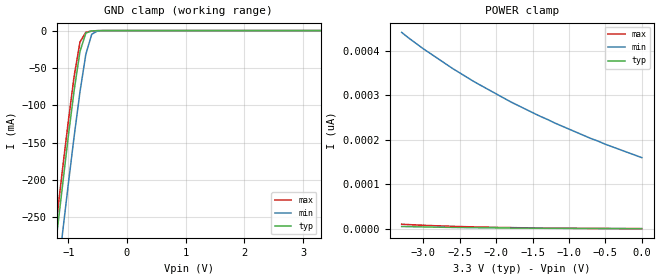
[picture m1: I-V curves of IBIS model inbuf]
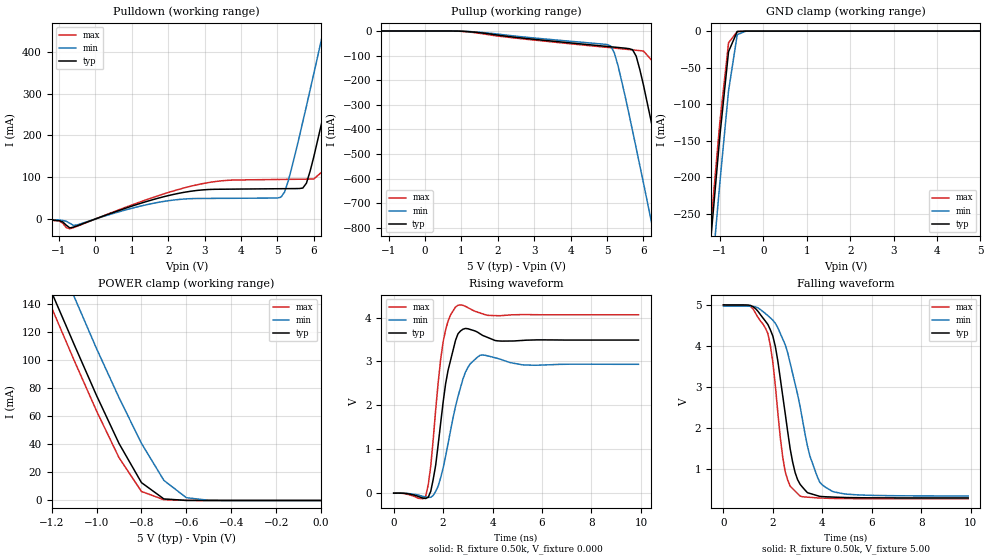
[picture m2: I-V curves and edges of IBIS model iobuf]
| IBIS file 64245l.ibs created by s2ibis2 version 1.0
| North Carolina State University Electronics Research Laboratory  1995
[IBIS ver]   2.1
[File name]   64245l.ibs
[File Rev]   0.1
[Date]   Friday, August 15, 1997
[Source]   IDT
[Notes]   1. Temp typ=25C, min=100C, max=0C 2. Ramp rates based on 500
   ohm load
[Copyright]   Copyright 1997, Integrated Device Technology, Inc.
[Disclaimer] Integrated Device Technology, Inc. ("IDT") hereby grants the
   user of this IBIS model a non-exclusive, nontransferable
   license to use this IBIS model under the following terms.
   The user is granted this license only to use the IBIS model
   and is not granted rights to sell, copy (except as needed to
   run the IBIS model), rent, lease or sub-license the IBIS model
   in whole or in part, or in modified form to anyone.
   The User may modify the IBIS model to suit its specific
   applications, but rights to derivative works and such
   modifications shall belong to IDT.
   This IBIS model is provided on an "AS IS" basis and IDT
   makes absolutely no warranty with respect to the information
   contained herein. IDT DISCLAIMS AND CUSTOMER WAIVES ALL
   WARRANTIES, EXPRESS AND IMPLIED, INCLUDING WARRANTIES OF
   MERCHANTABILITY AND FITNESS FOR A PARTICULAR PURPOSE. THE
   ENTIRE RISK AS TO QUALITY AND PERFORMANCE IS WITH THE
   USER ACCORDINGLY, IN NO EVENT SHALL IDT BE LIABLE
   FOR ANY DIRECT OR INDIRECT DAMAGES, WHETHER IN CONTRACT OR
   TORT, INCLUDING ANY LOST PROFITS OR OTHER INCIDENTAL,
   CONSEQUENTIAL, EXEMPLARY, OR PUNITIVE DAMAGES ARISING OUT OF
   THE USE OR APPLICATION OF THE IBIS model.  Further, IDT
   reserves the right to make changes without notice to any
   product herein to improve reliability, function, or design.
   IDT does not convey any license under patent rights or
   any other intellectual property rights, including those of
   third parties. IDT is not obligated to provide maintenance
   or support for the licensed IBIS model.
|   Component IDT54/74FCT164245/A/C
[Component]   IDT54/74FCT164245/A/C
[Manufacturer]   Integrated Device Technology Inc.
[Package]
| Following package parameters are for SO48-2(TSSOP) package
|[Package]
|| variable   typ   min   max
R_pkg   15.00m   10.00m   20.00m
L_pkg   2.30nh   1.40nh   4.50nH
C_pkg   0.40pF   0.35pF   0.60pF
| Following package parameters are for SO48-1(SSOP), E48-1(CERPAK) packages
|[Package]
|| variable   typ   min   max
|R_pkg   15.00m   10.00m   20.00m
|L_pkg   2.90nH   1.50nH   5.60nH
|C_pkg   0.40pF   0.26pF   0.50pF
[Pin]  signal_name   model_name   R_pin   L_pin   C_pin
1   1DIR   inbuf
2   1B1   iobuf
3   1B2   iobuf
4   GND   GND
5   1B3   iobuf
6   1B4   iobuf
7   VCC   POWER
8   1B5   iobuf
9   1B6   iobuf
10   GND   GND
11   1B7   iobuf
12   1B8   iobuf
13   2B1   iobuf
14   2B2   iobuf
15   GND   GND
16   2B3   iobuf
17   2B4   iobuf
18   VCC   POWER
19   2B5   iobuf
20   2B6   iobuf
21   GND   GND
22   2B7   iobuf
23   2B8   iobuf
24   2DIR   inbuf
25   2OEB   inbuf
26   2A8   iobuf
27   2A7   iobuf
28   GND   GND
29   2A6   iobuf
30   2A5   iobuf
31   VCC   POWER
32   2A4   iobuf
33   2A3   iobuf
34   GND   GND
35   2A2   iobuf
36   2A1   iobuf
37   1A8   iobuf
38   1A7   iobuf
39   GND   GND
40   1A6   iobuf
41   1A5   iobuf
42   VCC   POWER
43   1A4   iobuf
44   1A3   iobuf
45   GND   GND
46   1A2   iobuf
47   1A1   iobuf
48   1OEB   inbuf
| Models and submodels in the file (2): inbuf (Input), iobuf (I/O)
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| in   IN1   dummy_model
| oe   OE1   dummy_model
|   Model inbuf
[Model]   inbuf
Model_type   Input
Vinl =  0.800V
Vinh =  2.000V
C_comp   3.00pF   NA   NA
[Temperature Range]   25.00   100.00   0.000
[Voltage Range]   3.30V   3.00V   3.60V
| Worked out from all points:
|   GND clamp passes 1 mA (typ) near -0.62 V on its own axis
[GND_clamp]
| voltage   I(typ)   I(min)   I(max)
-3.3V     -1.781A    -1.841A    -1.762A
-1.3V     -346mA     -410mA     -324mA
-1.2V     -276mA     -341mA     -255mA
-1.1V     -209mA     -273mA     -187mA
-1V       -142mA     -206mA     -122mA
-900mV    -80.26mA   -142mA     -61.07mA
-800mV    -27.87mA   -81.82mA   -15.26mA
-700mV    -3.289mA   -31.47mA   -2.24mA
-600mV    -480uA     -4.848mA   -551uA
-500mV    -82.77uA   -464uA     -85.69uA
3.3V      588fA      178pA      482fA
[POWER_clamp]
| voltage   I(typ)   I(min)   I(max)
-3.3V     5.432pA    441pA      10.51pA
-3V       4.444pA    404pA      8.155pA
-2.6V     3.398pA    360pA      5.808pA
-2.3V     2.779pA    330pA      4.5pA
-1.8V     1.984pA    285pA      2.938pA
-1.2V     1.325pA    238pA      1.756pA
-700mV    945fA      203pA      1.142pA
0V        588fA      160pA      625fA
|   Model iobuf
[Model]   iobuf
Model_type   I/O
Polarity   Non-Inverting
Enable   Active-High
Vinl =  0.800V
Vinh =  2.000V
C_comp   3.00pF   NA   NA
[Temperature Range]   25.00   100.00   0.000
[Voltage Range]   5.00V   4.50V   5.50V
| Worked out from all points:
|   slope of the pulldown table from 0 to 0.75 V, typ, clamps not added: 32 ohm
|   slope of the pullup table from 0 to 0.75 V, typ, clamps not added: 16.9 kohm
|   GND clamp passes 1 mA (typ) near -0.60 V on its own axis
|   POWER clamp passes 1 mA (typ) near -0.69 V on its own axis
|   rising waveform, R_fixture 0.50k, V_fixture 0.000: 20-80 % time 485ps typ, 669ps min, 420ps max; typ from 0 V to 3.49 V
|   falling waveform, R_fixture 0.50k, V_fixture 5.00: 20-80 % time 708ps typ, 1.04ns min, 535ps max; typ from 5 V to 0.294 V
[Pulldown]
| voltage   I(typ)   I(min)   I(max)
-5V       0A         0A         0A
-1.4V     -1.4mA     -1.2mA     -1.5mA
-700mV    -21.48mA   -10.28mA   -23.37mA
2.4V      63.27mA    47.55mA    73.49mA
5.1V      72.54mA    52.22mA    94.74mA
5.3V      72.68mA    90.95mA    94.95mA
5.8V      85.74mA    270mA      95.45mA
6.4V      298mA      503mA      126mA
6.8V      454mA      660mA      272mA
7.2V      613mA      818mA      428mA
7.6V      772mA      977mA      586mA
10V       1.734A     1.934A     1.549A
[Pullup]
| voltage   I(typ)   I(min)   I(max)
-5V       0A         0A         0A
900mV     -315uA     -296uA     -632uA
5V        -62.63mA   -55.04mA   -66.48mA
5.2V      -65.46mA   -88.64mA   -69.4mA
5.7V      -75.8mA    -405mA     -76.67mA
5.8V      -102mA     -475mA     -78.12mA
6V        -219mA     -617mA     -81.11mA
6.4V      -498mA     -906mA     -148mA
6.8V      -787mA     -1.197A    -417mA
7.2V      -1.079A    -1.49A     -705mA
7.6V      -1.373A    -1.784A    -998mA
10V       -3.151A    -3.558A    -2.774A
[GND_clamp]
| voltage   I(typ)   I(min)   I(max)
-5V       -3.126A    -3.162A    -3.124A
-1.4V     -422mA     -485mA     -404mA
-1.2V     -280mA     -344mA     -261mA
-1V       -144mA     -208mA     -125mA
-800mV    -28.18mA   -82.09mA   -16.01mA
-600mV    -487uA     -4.87mA    -593uA
-400mV    -1.041uA   -20.98uA   -995nA
5V        1.904pA    145uA      2.071pA
[POWER_clamp]
| voltage   I(typ)   I(min)   I(max)
-5V       1.658A     1.682A     1.65A
-1.3V     186mA      220mA      175mA
-1.2V     148mA      182mA      137mA
-1.1V     111mA      145mA      99.7mA
-1V       74.62mA    108mA      63.64mA
-900mV    40.55mA    73.19mA    30.44mA
-800mV    12.71mA    40.62mA    6.427mA
-700mV    1.113mA    14.29mA    552uA
-600mV    55.94uA    1.985mA    66.61uA
-500mV    1.923uA    144uA      3.688uA
0V        1.904pA    260pA      3.223pA
[Ramp]
| variable   typ   min   max
dV/dt_r   2.09/0.49n   1.76/0.67n   2.44/0.42n
dV/dt_f   2.82/0.71n   2.52/1.02n   3.12/0.54n
R_load = 0.50k
[Rising Waveform]
R_fixture = 0.50k
V_fixture = 0.000
| time   V(typ)   V(min)   V(max)
0s        0V         0V         0V
1.3ns     -121mV     -88.65mV   -60.88mV
1.5ns     42.72mV    -93.72mV   620mV
1.6ns     317mV      -50.98mV   1.228V
1.8ns     1.107V     161mV      2.515V
2ns       2.073V     572mV      3.447V
2.5ns     3.477V     1.974V     4.239V
2.9ns     3.751V     2.754V     4.255V
3.5ns     3.627V     3.142V     4.102V
9.9ns     3.487V     2.935V     4.063V
[Falling Waveform]
R_fixture = 0.50k
V_fixture = 5.00
| time   V(typ)   V(min)   V(max)
0s        5V         4.97V      5V
1.1ns     4.987V     4.968V     4.961V
1.9ns     4.392V     4.684V     4.006V
2.1ns     3.989V     4.553V     3.035V
2.5ns     2.351V     4.03V      930mV
2.8ns     1.17V      3.328V     520mV
3.1ns     628mV      2.529V     340mV
3.8ns     349mV      807mV      295mV
4.4ns     315mV      456mV      282mV
9.9ns     294mV      341mV      275mV
